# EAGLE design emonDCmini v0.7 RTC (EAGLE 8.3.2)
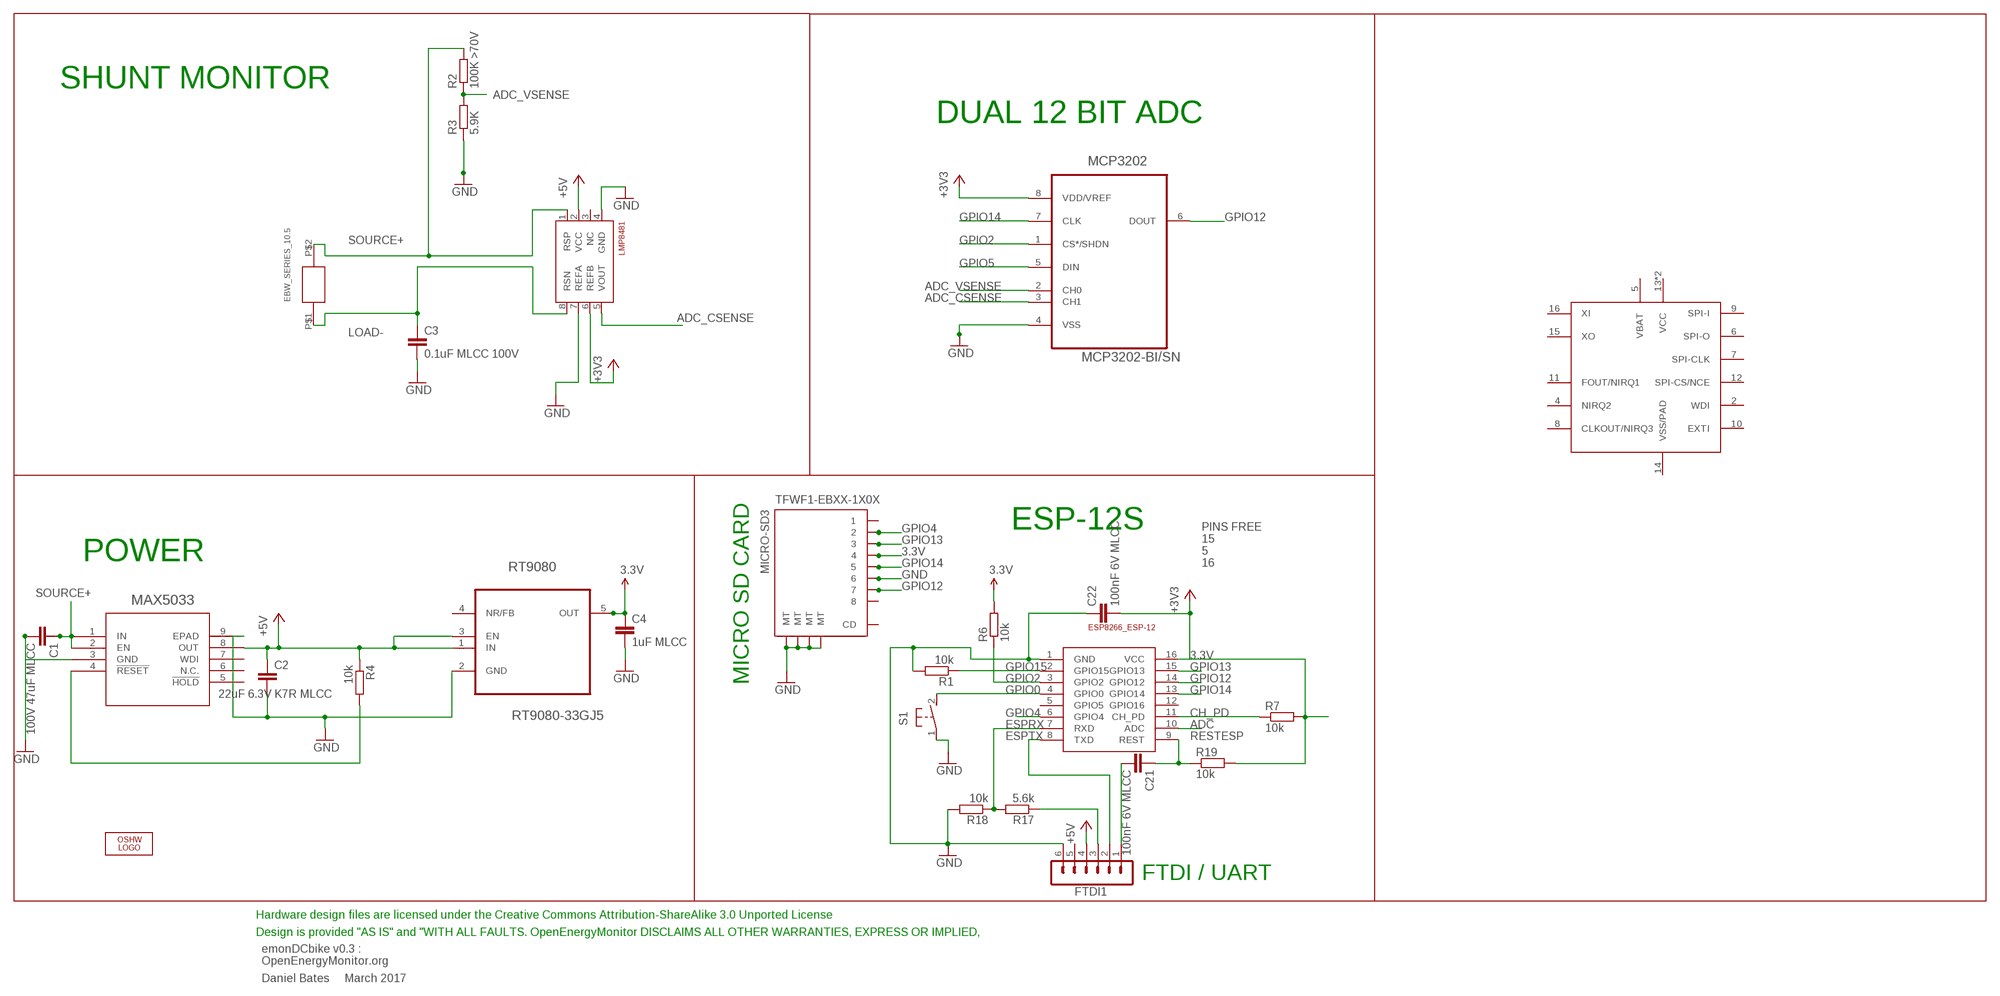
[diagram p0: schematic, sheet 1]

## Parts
C1  100V 47uF MLCC  C-EUC1206  [C1206]
C2  22uF 6.3V K7R MLCC  C-EUC1206  [C1206]
C3  0.1uF MLCC 100V  C-EUC0603  [C0603]
C4  1uF MLCC  C-EUC0603  [C0603]
C21  100nF 6V MLCC  C-EUC0603  [C0603]
C22  100nF 6V MLCC  C-EUC0603  [C0603]
EBW_SERIES_10.5  EBW_SERIES_10.5MM  [EBW_SERIES_10.5MM]
ESP-12  ESP8266_ESP-12  [ESP8266-ESP12]
FTDI1  FTDI-ESP  MA06-1  [MA06-1]
LMP8481  LMP8481-H  LMP8481LMP8481-H  [S-PDSO-G08]
LOGO1  OSHW_LOGO_6MILX0200-NT  [OSHW_6X200_NOTEXT]
MAX5033  MAX5033BUSA+  [21-0111D_SBE-14]
MCP3202  MCP3202-BI/SN  [SOIC127P600X175-8N]
R1  10k  R-EU_R0603  [R0603]
R2  100K >70V  R-EU_R0603  [R0603]
R3  5.9K  R-EU_R0603  [R0603]
R4  10k  R-EU_R0603  [R0603]
R6  10k  R-EU_R0603  [R0603]
R7  10k  R-EU_R0603  [R0603]
R17  5.6k  R-EU_R0603  [R0603]
R18  10k  R-EU_R0603  [R0603]
R19  10k  R-EU_R0603  [R0603]
RT9080  RT9080-33GJ5  [TSOT-23-5]
RTC  AB0815_RTC  [QFN16]
S1  DTSM-3  [DTSM-3]
TFWF1-EBXX-1X0X  MICRO-SD3  [TF-MICRO-SD_PP3*]

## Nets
3.3V: C4.1 C22.2 ESP-12.16(VCC) LMP8481.6(REFB) MCP3202.8(VDD/VREF) R6.2 R7.2 R19.2 RT9080.5(OUT) TFWF1-EBXX-1X0X.4 ; supply symbol labelled +3V3
+5V: C2.1 FTDI1.4 MAX5033.8(OUT) R4.1 RT9080.1(IN) RT9080.3(EN)
ADC: ESP-12.10(ADC)
ADC_CSENSE: LMP8481.5(VOUT) MCP3202.3(CH1)
ADC_VSENSE: MCP3202.2(CH0) R2.1 R3.2
CH_PD: ESP-12.11(CH_PD) R7.1
ESPRX: ESP-12.7(RXD) R17.2 R18.1
ESPTX: ESP-12.8(TXD) FTDI1.2
GND [thin_power]: C1.2 C2.2 C3.2 C4.2 C22.1 ESP-12.1(GND) FTDI1.6 LMP8481.4(GND) LMP8481.7(REFA) MAX5033.3(GND) MAX5033.9(EPAD) MCP3202.4(VSS) R1.2 R3.1 R18.2 RT9080.2(GND) S1.1 TFWF1-EBXX-1X0X.6 TFWF1-EBXX-1X0X.MT1(MT) TFWF1-EBXX-1X0X.MT2(MT) TFWF1-EBXX-1X0X.MT3(MT) TFWF1-EBXX-1X0X.MT4(MT)
GPIO0: ESP-12.4(GPIO0) S1.2
GPIO2: ESP-12.3(GPIO2) MCP3202.1(CS*/SHDN) R6.1
GPIO4: ESP-12.6(GPIO4) TFWF1-EBXX-1X0X.2
GPIO5: MCP3202.5(DIN)
GPIO12: ESP-12.14(GPIO12) MCP3202.6(DOUT) TFWF1-EBXX-1X0X.7
GPIO13: ESP-12.15(GPIO13) TFWF1-EBXX-1X0X.3
GPIO14: ESP-12.13(GPIO14) MCP3202.7(CLK) TFWF1-EBXX-1X0X.5
GPIO15: ESP-12.2(GPIO15) R1.1
LOAD- [power]: C3.1 EBW_SERIES_10.5.P$1 LMP8481.8(RSN)
N$1: MAX5033.4(!RESET) R4.2
N$36: FTDI1.3 R17.1
RESTESP: C21.1 ESP-12.9(REST) R19.1
RST: C21.2 FTDI1.1
SOURCE+ [power]: C1.1 EBW_SERIES_10.5.P$2 LMP8481.1(RSP) MAX5033.1(IN) MAX5033.2(EN) R2.2
Unconnected: ESP-12.5(GPIO5) ESP-12.12(GPIO16) FTDI1.5 LMP8481.2(VCC) LMP8481.3(NC) MAX5033.5(!HOLD) MAX5033.6(N.C.) MAX5033.7(WDI) RT9080.4(NR/FB) RTC.2(WDI) RTC.4(NIRQ2) RTC.5(VBAT) RTC.6(SPI-O) RTC.7(SPI-CLK) RTC.8(CLKOUT/NIRQ3) RTC.9(SPI-I) RTC.10(EXTI) RTC.11(FOUT/NIRQ1) RTC.12(SPI-CS/NCE) RTC.13(VCC) RTC.14(VSS/PAD) RTC.15(XO) RTC.16(XI) RTC.PAD(VCC) TFWF1-EBXX-1X0X.1 TFWF1-EBXX-1X0X.8 TFWF1-EBXX-1X0X.CD

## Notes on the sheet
- SHUNT MONITOR
- DUAL 12 BIT ADC
- ESP-12S
- POWER
- PINS FREE
  15
  5
  16
- MAX5033
- MICRO SD CARD
- FTDI / UART
- Hardware design files are licensed under the Creative Commons Attribution-ShareAlike 3.0 Unported License
- Design is provided "AS IS" and "WITH ALL FAULTS. OpenEnergyMonitor DISCLAIMS ALL OTHER WARRANTIES, EXPRESS OR IMPLIED,
- emonDCbike v0.3 :
  OpenEnergyMonitor.org
- Daniel Bates     March 2017

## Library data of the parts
C1-C4 C21 C22 = rcl:C-EU: CAPACITOR, European symbol
EBW_SERIES_10.5 = EBW series shunt:EBW_SERIES_10.5MM
ESP-12 = ESP8266-ESP12:ESP8266_ESP-12
FTDI1 = JeeLabs:MA06-1: PIN HEADER
LMP8481 = lmp8481b:LMP8481: LMP8481MM-H/NOPB 100V/V
LOGO1 = ohw-logo:OSHW_LOGO_6MIL; OC_FARNELL: unknown
MAX5033 = MAX5033:MAX5033BUSA+: VOLTAGE REGULATOR 3.3V; MANUFACTURER_PART_NUMBER: MAX5033BUSA+; VENDOR: MAXIM
MCP3202 = Microchip-MCP3202-BI_SN:MCP3202-BI/SN: IC ADC 12BIT 2.7V 2CH SPI,SOIC-8; MPN: MCP3202-BI/SN; OC_FARNELL: 1196803; OC_NEWARK: 96K3721; PACKAGE: SOIC-8; SUPPLIER: Microchip
R1 R4 R6 R7 R17-R19 = rcl:R-EU_: RESISTOR, European symbol
R2 = rcl:R-EU_: RESISTOR, European symbol; MPN: MCWR06X1003FTL
R3 = rcl:R-EU_: RESISTOR, European symbol; MPN: MCWR06X5901FTL
RT9080 = TSOT-23-5 REGULATOR 3.3v:RT9080-33GJ5: Low-Dropout Regulator; OC_FARNELL: 2679852; PACKAGE: SOT-23-5
RTC = AB0815 RTC:AB0815_RTC
S1 = switch-tact:DTSM-3
TFWF1-EBXX-1X0X = TFWF1-EBXX-1X0X:MICRO-SD

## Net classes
1 power: width 1.016 mm
2 thin_power: width 0.254 mm

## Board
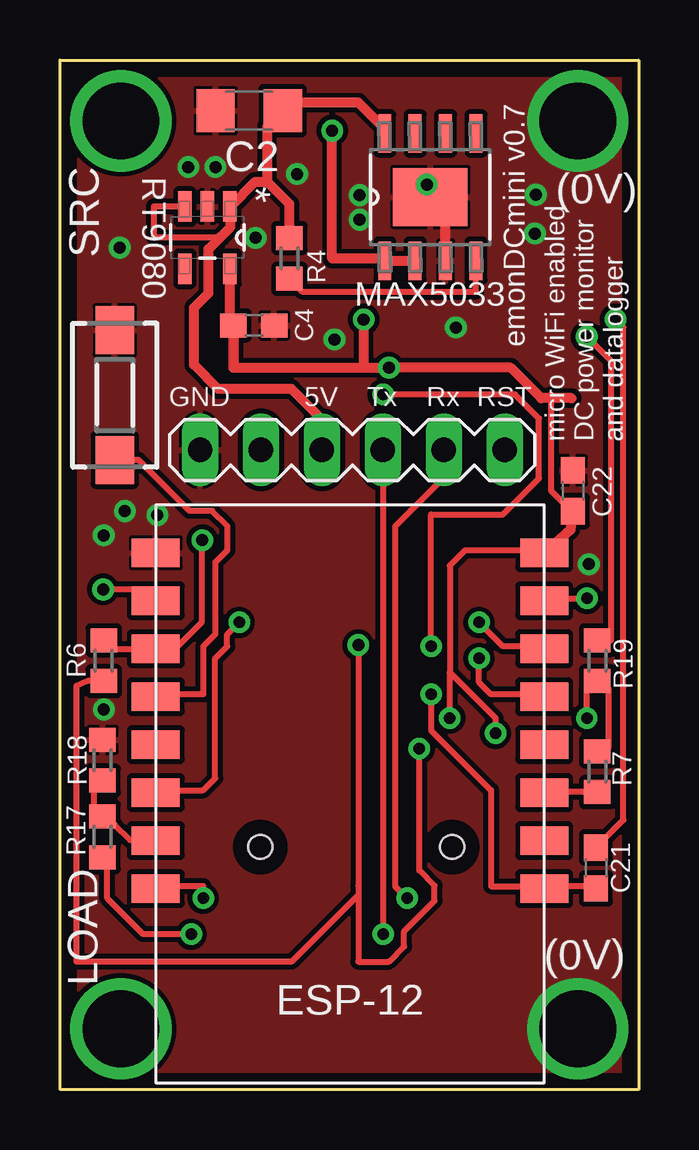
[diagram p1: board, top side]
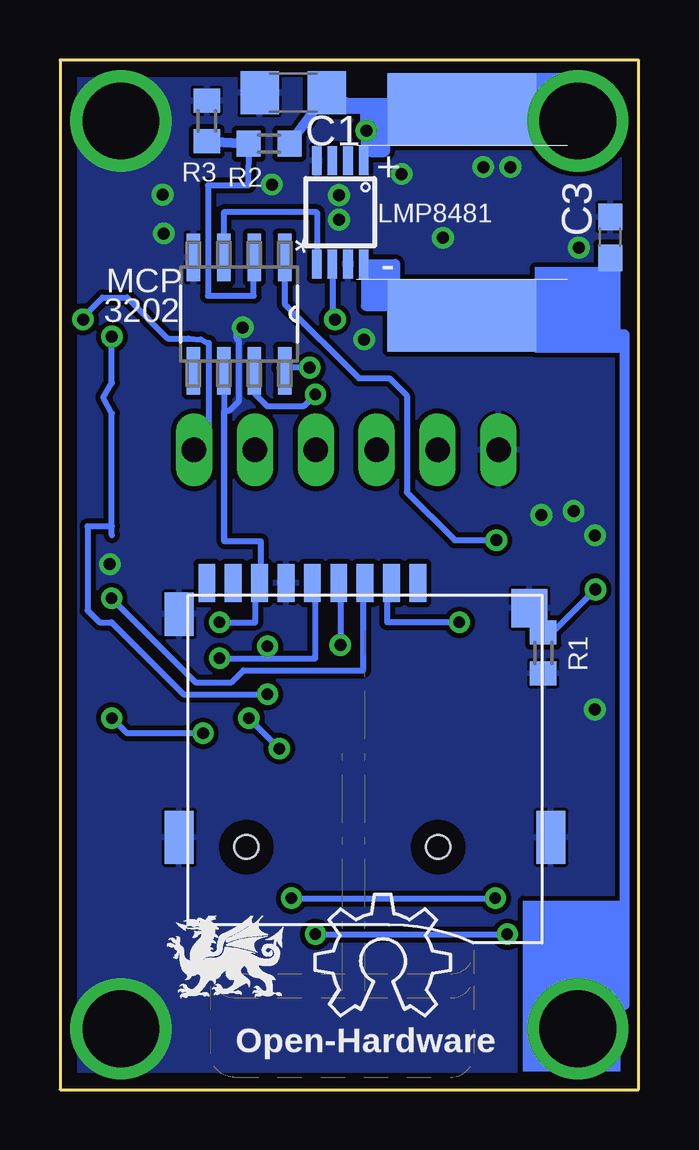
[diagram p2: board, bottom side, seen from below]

Size 24.13 x 42.93 mm. Coordinates in mm from the lower left corner, seen from the top.
Outline: 0,42.93 24.13,42.93 24.13,0 0,0 0,42.93
Copper layers (1*16): Top 0.035mm / dielectric 1.5mm / Bottom 0.035mm
Design rules "default *": minimum track width 10mil, minimum drill 19mil, track to track 8mil, track to pad 8mil, pad to pad 8mil, via to via 8mil, smd to smd 8mil, copper to edge 25mil, drill to drill 8mil, minimum pad ring 10mil, minimum via ring 8mil, stop-mask expansion 4mil, vias tented up to drill 0mil, thermal gap 5mil

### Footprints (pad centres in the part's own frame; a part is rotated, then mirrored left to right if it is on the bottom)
C1206 = smd 1.6 x 1.8: 1 -1.4,0; 2 1.4,0
C0603 = smd 1.1 x 1: 1 -0.85,0; 2 0.85,0
EBW_SERIES_10.5MM = smd 3 x 6.2: P$1 -4.3,0; P$2 4.3,0
ESP8266-ESP12 = smd 2 x 1.2: 1 16.2,2; 2 16.2,4; 3 16.2,6; 4 16.2,8; 5 16.2,10; 6 16.2,12; 7 16.2,14; 8 16.2,16; 9 0,16; 10 0,14; 11 0,12; 12 0,10; 13 0,8; 14 0,6; 15 0,4; 16 0,2
MA06-1 = drill 1.016 long: 1 0,0; 2 2.54,0; 3 5.08,0; 4 7.62,0; 5 10.16,0; 6 12.7,0
S-PDSO-G08 = smd 0.4 x 1.2: 1 -0.975,-2.157; 2 -0.325,-2.157; 3 0.325,-2.157; 4 0.975,-2.157; 5 0.975,2.157; 6 0.325,2.157; 7 -0.325,2.157; 8 -0.975,2.157
21-0111D_SBE-14 = smd 1.6 x 0.533: 1 -2.654,1.905; 2 -2.654,0.635; 3 -2.654,-0.635; 4 -2.654,-1.905; 5 2.654,-1.905; 6 2.654,-0.635; 7 2.654,0.635; 8 2.654,1.905 | smd 2.413 x 3.099: 9 0,0
SOIC127P600X175-8N = smd 1.981 x 0.559: 1 -2.362,1.905; 2 -2.362,0.635; 3 -2.362,-0.635; 4 -2.362,-1.905; 5 2.362,-1.905; 6 2.362,-0.635; 7 2.362,0.635; 8 2.362,1.905
R0603 = smd 1 x 1.1: 1 -0.85,0; 2 0.85,0
TSOT-23-5 = smd 1.27 x 0.559: 1 -1.295,0.94; 2 -1.295,0; 3 -1.295,-0.94; 4 1.295,-0.94; 5 1.295,0.94
QFN16 = smd 0.85 x 0.3: 1 -1.655,0.75; 2 -1.655,0.25; 3 -1.655,-0.25; 4 -1.655,-0.75; 9 1.655,-0.75; 10 1.655,-0.25; 11 1.655,0.25; 12 1.655,0.75 | smd 0.3 x 0.85: 5 -0.75,-1.655; 6 -0.25,-1.655; 7 0.25,-1.655; 8 0.75,-1.655; 13 0.75,1.655; 14 0.25,1.655; 15 -0.25,1.655; 16 -0.75,1.655 | smd 1.9 x 1.9: PAD 0,0
DTSM-3 = smd 2 x 1.6: 1 -2.7,0; 2 2.7,0
TF-MICRO-SD_PP3* = smd 0.7 x 1.6: 1 2.2,11; 2 1.1,11; 3 0,11; 4 -1.1,11; 5 -2.2,11; 6 -3.3,11; 7 -4.4,11; 8 -5.5,11; CD -6.6,11 | smd 1.2 x 2.2: MT1 -7.75,0.4; MT2 7.75,0.4 | smd 1.2 x 1.8: MT3 -7.75,9.7 | smd 1.5 x 1.6: MT4 6.85,9.95 | hole 1: -4.95,0; 3.05,0

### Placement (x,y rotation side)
C1  14.4,41.56 180 bottom
C2  7.89,40.81 180 top
C3  1.19,35.53 90 bottom
C4  8.09,31.86 0 top
C21  22.35,9.25 90 top
C22  21.39,24.97 270 top
EBW_SERIES_10.5  7.37,36.58 90 bottom
ESP-12  20.19,24.38 180 top
FTDI1  18.54,26.67 180 top
LMP8481  12.45,36.58 180 bottom
LOGO1  13.5,3.07 0 bottom
MAX5033  15.44,37.21 90 top
MCP3202  16.66,32.33 270 bottom
R1  3.98,18.21 270 bottom
R2  15.41,39.44 0 bottom
R3  18,40.38 270 bottom
R4  9.57,34.66 270 top
R6  1.83,17.88 270 top
R7  22.4,13.26 90 top
R17  1.78,10.54 90 top
R18  1.78,13.74 90 top
R19  22.4,17.88 270 top
RT9080  6.15,35.52 270 top
RTC  not placed on the board
S1  2.29,28.96 270 top
TFWF1-EBXX-1X0X  11.41,10.12 0 bottom
U$3  [DRAGON_LOGO_NOTEXT]  17.07,5.51 0 bottom

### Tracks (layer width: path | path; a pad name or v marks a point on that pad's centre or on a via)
3.3V  (via drill 0.48, 0.5)
  Top 0.254: R19.2 | 21.97,14.22 R7.2 22.86,14.22 22.86,16.76 R19.2 | R6.2 1.13,17.03 0.69,16.84 0.69,5.33 9.65,5.33 12.44,8.12 12.44,8.51 | C22.2 20.98,24.48 20.48,24.98 20.48,28.98 20.48,28.83 | v12.44,18.54 12.44,8.51 | v21.97,15.49 21.97,16.76 R19.2 | v18.16,14.86 18.16,15.49 16.26,17.4 | 16.26,17.4 16.26,21.84 16.89,22.48 20.07,22.48 ESP-12.16 | v16.26,15.49 16.26,17.4 | v14.99,14.22 14.99,9.14 15.62,8.51 15.62,7.87 14.35,6.6 14.35,5.97 13.72,5.33 12.45,5.33 12.45,8.51 12.44,8.51
  Top 0.406: C22.2 21.29,23.35 ESP-12.16 | 21.34,28.83 20.48,28.83 20.07,28.82 18.8,30.1 v13.72,30.1 12.66,30.1 | 7.24,30.11 | 7.24,30.11 C4.1 | C4.1 7.09,31.86 RT9080.5 | v12.66,32.11 12.66,30.1 | C4.1 7.24,30.1 12.66,30.1
  Bottom 0.254: v13.72,30.1 14.99,30.1 MCP3202.8 | LMP8481.6 12.77,32.22 | TFWF1-EBXX-1X0X.4 12.44,21.12 v12.44,18.54 | v21.97,15.49 21.34,14.86 v18.16,14.86 | v14.99,14.22 v16.26,15.49
  Bottom 0.406: 12.77,32.22 v12.66,32.11
+5V
  Top 0.254: 6.69,35.54 6.69,35.55 3.91,35.55 3.91,36.82 RT9080.3
  Top 0.406: FTDI1.4 10.92,27.94 9.65,29.21 6.6,29.21 5.59,30.23 5.59,32.6 6.2,33.2 6.2,35.05 6.69,35.54 7.11,35.96 | 9.29,41.05 C2.1 | R4.1 9.57,36.92 8.64,37.85 | RT9080.1 7.11,36.82 8.14,37.85 8.64,37.85 | MAX5033.8 13.54,40.1 13.49,40.1 12.45,41.15 9.62,41.15 C2.1 | C2.1 8.64,40.16 8.64,37.85
  Top 0.424: 7.11,35.96 7.11,36.82
ADC_CSENSE
  Bottom 0.254: MCP3202.3 17.3,36.58 13.42,36.58 LMP8481.5
ADC_VSENSE
  Bottom 0.254: 16,34.7 MCP3202.2 16.05,34.7 16.05,33.1 17.96,33.1 17.96,37.69 16.29,37.69 R2.1
  Bottom 0.406: R3.2 R2.1
CH_PD
  Top 0.254: R7.1 20.32,12.41 ESP-12.11
ESPRX
  Top 0.254: 4.11,10.38 arc90 ESP-12.7 | 3.56,10.41 3.97,10.41 ESP-12.7 | 1.9,11.37 R17.2 | R18.1 1.75,12.79 1.43,12.48 1.43,11.37 1.75,11.37 R17.2 | 3.56,10.41 2.92,10.41 2.29,11.05 R17.2 | 3.56,10.41 ESP-12.7
ESPTX  (via drill 0.48)
  Top 0.254: v5.98,7.98 5.98,8.48 4.48,8.48 ESP-12.8 | v14.48,7.98 13.98,8.48 13.98,23.48 15.98,25.48 15.98,26.48 FTDI1.2
  Bottom 0.254: v14.48,7.98 v5.98,7.98
GND  (via drill 0.5, 3.2)
  Top 0.254: ESP-12.1 4.19,22.48 4.22,22.29
  Top 0.406: MAX5033.3 16.08,36.58
  Bottom 0.254: 17.28,22.86 17.28,28.32 17.05,28.32 16.66,28.71 16.66,31.21 16.76,31.31 16.76,31.75
  other vias: 19.84,37.31 1.83,15.85 2.71,24.13 4.06,23.96 16.51,31.78 9.88,38.18 12.5,37.29 11.45,31.28 21.59,2.54 21.59,40.39 22.05,21.91 15.29,37.74 6.48,38.46 12.5,36.27 1.82,23.11 19.8,35.7 5.35,38.46 2.49,35.1 8.16,35.51
  pour Top: 0.25,42.67 23.88,42.67 23.88,0.25 0.25,0.25
  pour Bottom: 0.25,42.67 23.88,42.67 23.88,0.25 0.25,0.25
GPIO0
  Top 0.254: S1.2 3.28,26.26 5.4,24.13 6.35,24.13 6.96,23.52 6.98,23.48 6.98,22.48 6.48,21.98 6.48,18.98 5.98,18.48 5.98,16.48 4.48,16.48 ESP-12.4
GPIO2  (via drill 0.5)
  Top 0.254: R6.1 1.84,18.38 ESP-12.3 4.8,18.38 5.92,19.5 5.92,23.15 v5.93,22.91
  Bottom 0.254: MCP3202.1 14.76,32.75 11.67,29.66 10.39,29.66 9.66,28.94 9.66,24.91 7.67,22.91 v5.93,22.91
GPIO4  (via drill 0.48)
  Top 0.254: v7.48,19.48 6.98,18.98 6.98,18.48 6.48,17.98 6.48,12.98 5.98,12.48 4.48,12.48 ESP-12.6
  Bottom 0.254: v7.48,19.48 10.48,19.48 10.48,20.98 TFWF1-EBXX-1X0X.2
GPIO12  (via drill 0.48)
  Top 0.254: v17.48,19.48 18.48,18.48 19.98,18.48 ESP-12.14
  Bottom 0.254: v17.48,19.48 15.98,19.48 15.98,20.98 TFWF1-EBXX-1X0X.7 15.75,21.12 15.75,22.86 17.26,22.86 17.26,29.08 17.3,29.08 MCP3202.6
GPIO13  (via drill 0.48)
  Top 0.254: v21.98,20.48 20.48,20.48 ESP-12.15
  Bottom 0.254: v21.98,20.48 18.48,16.98 16.98,16.98 16.48,17.48 11.48,17.48 11.48,20.98 TFWF1-EBXX-1X0X.3
GPIO14  (via drill 0.48)
  Top 0.254: v17.48,17.98 17.48,16.98 17.98,16.48 19.98,16.48 ESP-12.13 | v13.48,28.98 18.98,28.98 19.98,27.98 19.98,25.48 18.48,23.98 15.48,23.98 v15.48,18.48
  Bottom 0.254: v17.48,17.98 15.48,17.98 | 15.48,17.98 13.48,17.98 13.48,20.98 TFWF1-EBXX-1X0X.5 | v13.48,28.98 13.98,28.48 15.48,28.48 15.98,28.98 15.98,29.48 MCP3202.7 | 15.48,17.98 v15.48,18.48
GPIO15  (via drill 0.5)
  Top 0.254: ESP-12.2 3.52,20.85 v1.8,20.85
  Bottom 0.254: v1.8,20.85 3.59,19.06 R1.1
LOAD-  (via drill 3.2)
  Bottom 0.254: 11.43,34.29 11.47,34.33 LMP8481.8
  Bottom 0.406: 1.2,31.5 6.59,31.5 EBW_SERIES_10.5.P$1 7.37,33.27 10.16,33.27 10.16,34.42 LMP8481.8 | 1.2,31.5 0.58,31.5 0.58,3.53 2.54,3.53 v2.54,2.54 | 11.43,34.29 11.37,34.31 11.37,32.67 10.28,32.65 10.28,32.66 10.34,32.66 10.34,34.17 11.19,34.17 11.19,34.18 11.18,34.18 11.18,32.99 10.55,32.99 10.55,32.94 10.59,32.94 10.59,33.92 10.87,33.92 10.87,33.96 10.89,33.96 10.89,33.23 | C3.1 1.2,34.68 1.2,31.5
N$1
  Top 0.254: R4.2 10.1,33.27 17.35,33.27 MAX5033.4
N$36  (via drill 0.48)
  Top 0.254: v5.48,6.48 3.48,6.48 1.98,7.98 1.98,9.48 R17.1 | v13.48,6.48 13.48,26.48 FTDI1.3
  Bottom 0.254: v13.48,6.48 v5.48,6.48
RESTESP  (via drill 0.48, 0.5)
  Top 0.254: C21.1 21.97,8.51 20.7,8.51 ESP-12.9 19.98,8.48 17.98,8.48 17.98,12.48 15.48,14.98 v15.48,16.48 | R19.1 22.99,18.73 22.99,30.37 v21.97,31.39
  Bottom 0.254: v21.97,31.39 21.97,29.46 22.33,28.85 21.97,28.19 21.97,23.48 | 21.97,23.11 21.97,23.48 | v15.48,16.48 18.98,16.48 21.98,19.48 22.48,19.48 22.98,19.98 22.98,23.48 21.97,23.48
RST  (via drill 0.5)
  Top 0.254: C21.2 23.49,11.24 23.49,31.78 v23.17,32.11
  Bottom 0.254: v23.17,32.11 23.17,32.2 22.35,33.02 21.34,33.02 19.63,31.32 18.77,31.32 18.25,31.28 17.97,31.12 17.93,31.12 17.93,26.67 FTDI1.1
SOURCE+  (via drill 0.5, 3.2)
  Top 0.406: MAX5033.1 13.54,34.59 | v11.35,39.98 11.35,34.65 13.54,34.65 MAX5033.1 | MAX5033.1 MAX5033.2
  Bottom 0.254: v11.35,39.98 11.47,40.02 | 11.47,40.02 LMP8481.1 | 11.49,40.85 11.49,40.02 | 11.49,40.02 11.49,39.94 11.43,39.88 | 11.2,40.99 11.34,40.85 11.49,40.85 | 11.49,40.87 11.49,40.85 | 11.47,40.02 11.49,40.02
  Bottom 0.406: 7.37,41.63 EBW_SERIES_10.5.P$2 7.37,39.62 10.66,39.62 10.66,39.63 | 2.29,40.89 2.54,40.89 v2.54,40.39 | R2.2 C1.1 11.49,40.85 | 10.16,41.15 12.7,41.15 12.7,40.89 10.67,40.89 10.66,41.02
  Bottom 0.61: 10.66,41.02 10.66,39.63 10.67,39.16 11.1,39.16 11.1,40.89 11.2,40.99
  Bottom 1.016: 2.29,40.89 7.37,40.89 EBW_SERIES_10.5.P$2
(copper drawn outside any net)
  shapes: Bottom area x3

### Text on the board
bPlace: Open-Hardware
tNames: (0V) | SRC | emonDCmini v0.7 | GND | 5V | Tx | Rx | RST | micro WiFi enabled / DC power monitor / and datalogger | LOAD | (0V)
bNames: MCP | 3202
_tsilk: Designed in | North Wales | Made in UK
_bsilk: SMT V0.6 rev3 | emonTx | wireless energy monitoring node | SMT V0.6 rev3 | emonTx | SMT V0.6 rev3 | emonTx | Technology that helps us live within ecological limits | wireless energy monitoring node | wireless energy monitoring node | Designed in North Wales UK by Glyn Hudson & Trystan Lea | Technology that helps us live within ecological limits | Technology that helps us live within ecological limits | Designed in North Wales UK by Glyn Hudson & Trystan Lea | 165mm ant | 433Mhz | Designed in North Wales UK by Glyn Hudson & Trystan Lea | 165mm ant | 165mm ant | 433Mhz | 433Mhz | 868Mhz | 82mm ant | 82mm ant | 82mm ant | 868Mhz | 868Mhz | 78mm ant | 915Mhz | 78mm ant | 915Mhz | 78mm ant | 915Mhz | 165mm ant | 433Mhz | 82mm ant | 868Mhz | 78mm ant | 915Mhz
